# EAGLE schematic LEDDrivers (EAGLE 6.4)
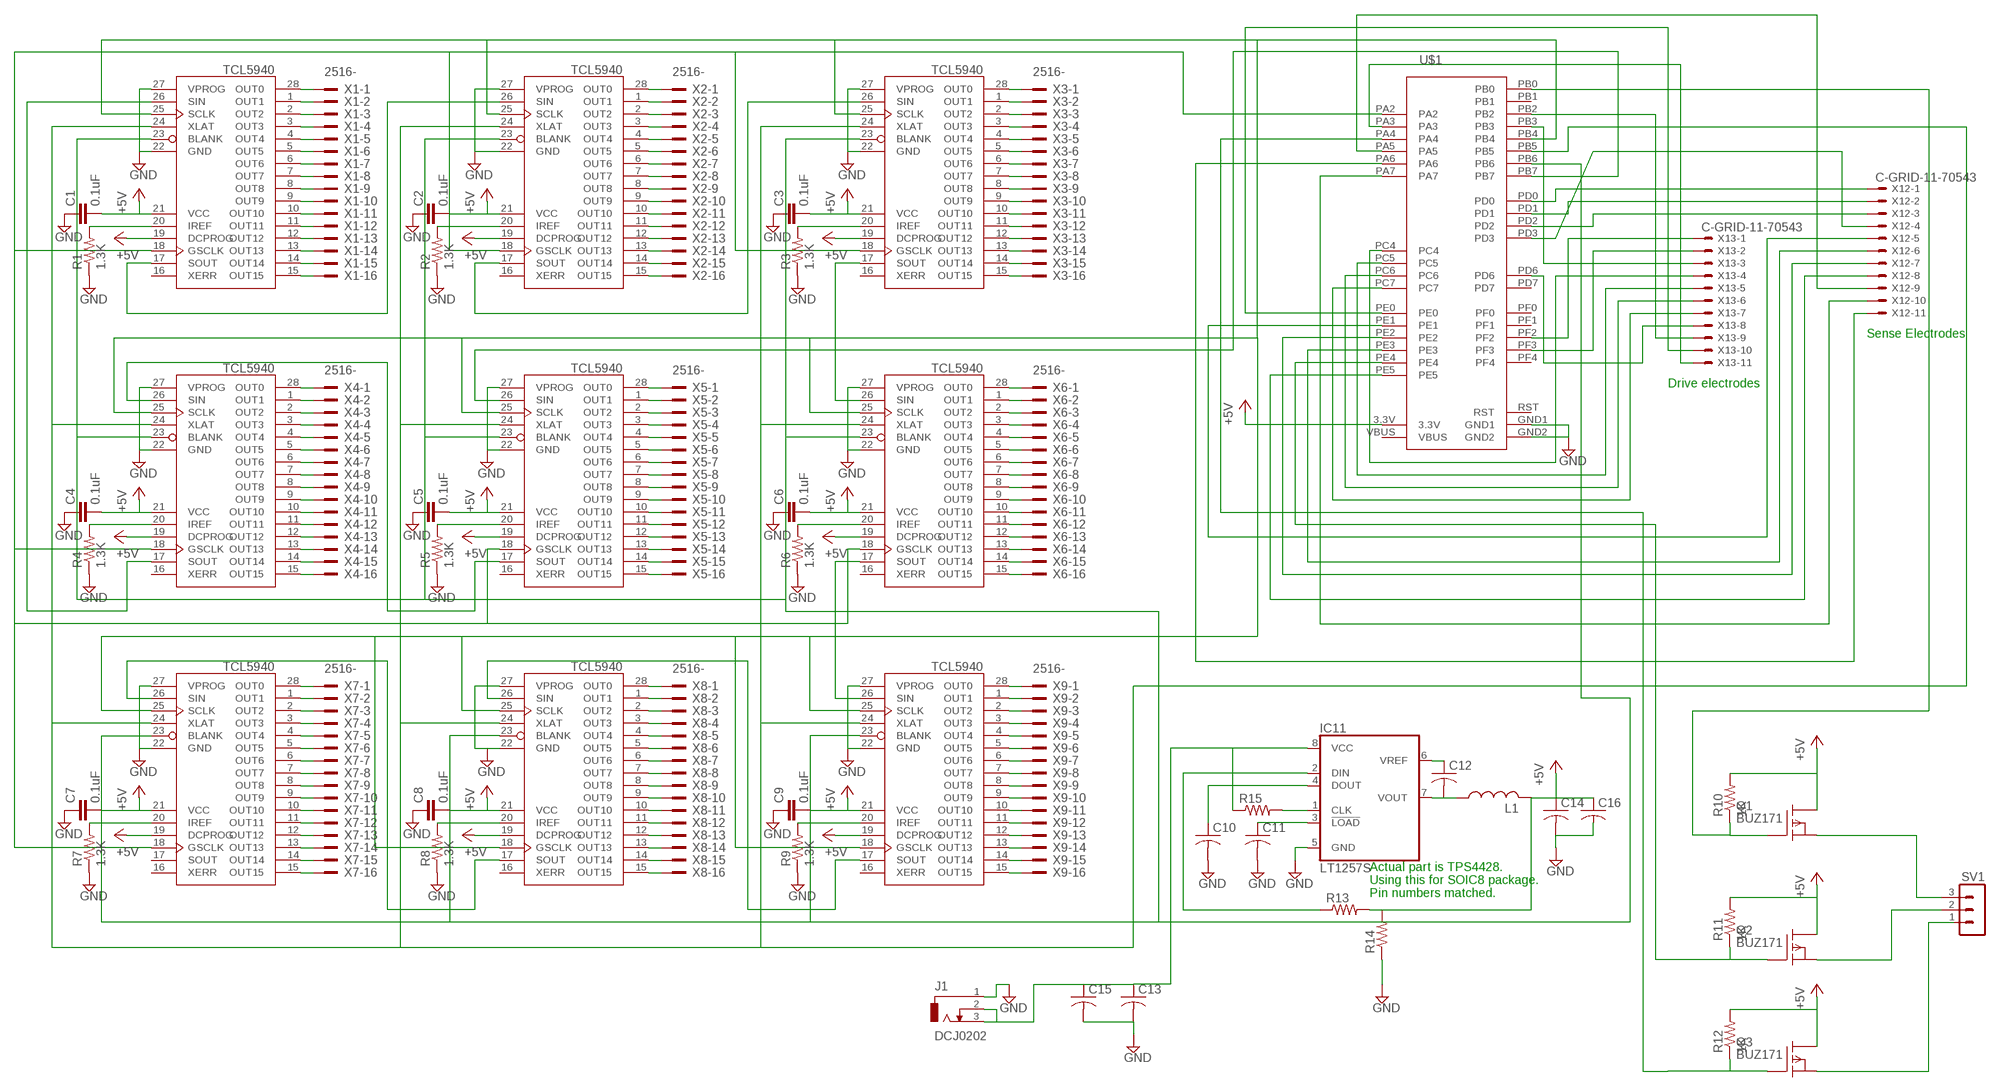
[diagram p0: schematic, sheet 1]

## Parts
C1  0.1uF  C-EU025-024X044  [C025-024X044]
C2  0.1uF  C-EU025-024X044  [C025-024X044]
C3  0.1uF  C-EU025-024X044  [C025-024X044]
C4  0.1uF  C-EU025-024X044  [C025-024X044]
C5  0.1uF  C-EU025-024X044  [C025-024X044]
C6  0.1uF  C-EU025-024X044  [C025-024X044]
C7  0.1uF  C-EU025-024X044  [C025-024X044]
C8  0.1uF  C-EU025-024X044  [C025-024X044]
C9  0.1uF  C-EU025-024X044  [C025-024X044]
C10  C-US025-024X044  [C025-024X044]
C11  C-US025-024X044  [C025-024X044]
C12  C-US025-024X044  [C025-024X044]
C13  C-US025-024X044  [C025-024X044]
C14  C-US025-024X044  [C025-024X044]
C15  C-US025-024X044  [C025-024X044]
C16  C-US025-024X044  [C025-024X044]
IC1  TCL5940  [DIP28]
IC2  TCL5940  [DIP28]
IC3  TCL5940  [DIP28]
IC4  TCL5940  [DIP28]
IC5  TCL5940  [DIP28]
IC6  TCL5940  [DIP28]
IC7  TCL5940  [DIP28]
IC8  TCL5940  [DIP28]
IC9  TCL5940  [DIP28]
IC11  LT1257S  [SOIC8]
J1  DCJ0202  [DCJ0202]
L1  L-US0207/7  [0207/7]
Q1  BUZ171  [TO220]
Q2  BUZ171  [TO220]
Q3  BUZ171  [TO220]
R1  1.3K  R-US_0204/2V  [0204V]
R2  1.3K  R-US_0204/2V  [0204V]
R3  1.3K  R-US_0204/2V  [0204V]
R4  1.3K  R-US_0204/2V  [0204V]
R5  1.3K  R-US_0204/2V  [0204V]
R6  1.3K  R-US_0204/2V  [0204V]
R7  1.3K  R-US_0204/2V  [0204V]
R8  1.3K  R-US_0204/2V  [0204V]
R9  1.3K  R-US_0204/2V  [0204V]
R10  1K  R-US_0204/2V  [0204V]
R11  1K  R-US_0204/2V  [0204V]
R12  1K  R-US_0204/2V  [0204V]
R13  R-US_0204/5  [0204/5]
R14  R-US_0204/5  [0204/5]
R15  R-US_0204/5  [0204/5]
SV1  MA03-1  [MA03-1]
U$1  STELLARIS-LAUNCHPADSTELLARIS-LAUNCHPAD-XL  [LAUNCHPAD-XL]
X1  2516-  [PAK100/2500-16]
X2  2516-  [PAK100/2500-16]
X3  2516-  [PAK100/2500-16]
X4  2516-  [PAK100/2500-16]
X5  2516-  [PAK100/2500-16]
X6  2516-  [PAK100/2500-16]
X7  2516-  [PAK100/2500-16]
X8  2516-  [PAK100/2500-16]
X9  2516-  [PAK100/2500-16]
X12  C-GRID-11-70543  [70543-11]
X13  C-GRID-11-70543  [70543-11]

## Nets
+5V: C1.2 C2.2 C3.2 C4.2 C5.2 C6.2 C7.2 C8.2 C9.2 C14.1 C16.1 IC1.19(DCPROG) IC1.21(VCC) IC2.19(DCPROG) IC2.21(VCC) IC3.19(DCPROG) IC3.21(VCC) IC4.19(DCPROG) IC4.21(VCC) IC5.19(DCPROG) IC5.21(VCC) IC6.19(DCPROG) IC6.21(VCC) IC7.19(DCPROG) IC7.21(VCC) IC8.19(DCPROG) IC8.21(VCC) IC9.19(DCPROG) IC9.21(VCC) L1.2 Q1.2(D) Q2.2(D) Q3.2(D) R10.2 R11.2 R12.2 R13.2 R14.2 U$1.3.3V
GND: C1.1 C2.1 C3.1 C4.1 C5.1 C6.1 C7.1 C8.1 C9.1 C10.2 C11.2 C13.2 C14.2 C15.2 IC1.22(GND) IC1.27(VPROG) IC2.22(GND) IC2.27(VPROG) IC3.22(GND) IC3.27(VPROG) IC4.22(GND) IC4.27(VPROG) IC5.22(GND) IC5.27(VPROG) IC6.22(GND) IC6.27(VPROG) IC7.22(GND) IC7.27(VPROG) IC8.22(GND) IC8.27(VPROG) IC9.22(GND) IC9.27(VPROG) IC11.5(GND) J1.1 R1.1 R2.1 R3.1 R4.1 R5.1 R6.1 R7.1 R8.1 R9.1 R14.1 U$1.GND1 U$1.GND2
N$1: IC1.26(SIN) IC7.17(SOUT)
N$2: IC7.20(IREF) R1.2
N$3: IC1.20(IREF) R2.2
N$4: IC1.28(OUT0) X2.1
N$5: IC1.3(OUT3) X2.4
N$6: IC1.4(OUT4) X2.5
N$7: IC1.5(OUT5) X2.6
N$8: IC1.6(OUT6) X2.7
N$9: IC1.7(OUT7) X2.8
N$10: IC1.8(OUT8) X2.9
N$11: IC1.9(OUT9) X2.10
N$12: IC1.10(OUT10) X2.11
N$13: IC1.11(OUT11) X2.12
N$14: IC1.12(OUT12) X2.13
N$15: IC7.28(OUT0) X1.1
N$16: IC1.13(OUT13) X2.14
N$17: IC1.14(OUT14) X2.15
N$18: IC1.15(OUT15) X2.16
N$19: IC7.1(OUT1) X1.2
N$20: IC7.2(OUT2) X1.3
N$21: IC7.3(OUT3) X1.4
N$22: IC7.4(OUT4) X1.5
N$23: IC7.5(OUT5) X1.6
N$24: IC7.6(OUT6) X1.7
N$25: IC7.7(OUT7) X1.8
N$26: IC7.8(OUT8) X1.9
N$27: IC7.9(OUT9) X1.10
N$28: IC7.10(OUT10) X1.11
N$29: IC7.11(OUT11) X1.12
N$30: IC7.12(OUT12) X1.13
N$31: IC7.13(OUT13) X1.14
N$32: IC7.14(OUT14) X1.15
N$33: IC7.15(OUT15) X1.16
N$34: IC1.1(OUT1) X2.2
N$35: IC1.2(OUT2) X2.3
N$36: IC1.17(SOUT) IC2.26(SIN)
N$37: IC2.20(IREF) R3.2
N$38: IC2.28(OUT0) X3.1
N$39: IC2.3(OUT3) X3.4
N$40: IC2.4(OUT4) X3.5
N$41: IC2.5(OUT5) X3.6
N$42: IC2.6(OUT6) X3.7
N$43: IC2.7(OUT7) X3.8
N$44: IC2.8(OUT8) X3.9
N$45: IC2.9(OUT9) X3.10
N$46: IC2.10(OUT10) X3.11
N$47: IC2.11(OUT11) X3.12
N$48: IC2.12(OUT12) X3.13
N$49: IC2.13(OUT13) X3.14
N$50: IC2.14(OUT14) X3.15
N$51: IC2.15(OUT15) X3.16
N$52: IC2.1(OUT1) X3.2
N$53: IC2.2(OUT2) X3.3
N$54: IC2.17(SOUT) IC5.26(SIN)
N$55: IC3.20(IREF) R4.2
N$56: IC3.28(OUT0) X4.1
N$57: IC3.3(OUT3) X4.4
N$58: IC3.4(OUT4) X4.5
N$59: IC3.5(OUT5) X4.6
N$60: IC3.6(OUT6) X4.7
N$61: IC3.7(OUT7) X4.8
N$62: IC3.8(OUT8) X4.9
N$63: IC3.9(OUT9) X4.10
N$64: IC3.10(OUT10) X4.11
N$65: IC3.11(OUT11) X4.12
N$66: IC3.12(OUT12) X4.13
N$67: IC3.13(OUT13) X4.14
N$68: IC3.14(OUT14) X4.15
N$69: IC3.15(OUT15) X4.16
N$70: IC3.1(OUT1) X4.2
N$71: IC3.2(OUT2) X4.3
N$72: IC3.17(SOUT) IC7.26(SIN)
N$73: IC4.20(IREF) R5.2
N$74: IC4.28(OUT0) X5.1
N$75: IC4.3(OUT3) X5.4
N$76: IC4.4(OUT4) X5.5
N$77: IC4.5(OUT5) X5.6
N$78: IC4.6(OUT6) X5.7
N$79: IC4.7(OUT7) X5.8
N$80: IC4.8(OUT8) X5.9
N$81: IC4.9(OUT9) X5.10
N$82: IC4.10(OUT10) X5.11
N$83: IC4.11(OUT11) X5.12
N$84: IC4.12(OUT12) X5.13
N$85: IC4.13(OUT13) X5.14
N$86: IC4.14(OUT14) X5.15
N$87: IC4.15(OUT15) X5.16
N$88: IC4.1(OUT1) X5.2
N$89: IC4.2(OUT2) X5.3
N$90: IC3.26(SIN) IC4.17(SOUT)
N$91: IC5.20(IREF) R6.2
N$92: IC5.28(OUT0) X6.1
N$93: IC5.3(OUT3) X6.4
N$94: IC5.4(OUT4) X6.5
N$95: IC5.5(OUT5) X6.6
N$96: IC5.6(OUT6) X6.7
N$97: IC5.7(OUT7) X6.8
N$98: IC5.8(OUT8) X6.9
N$99: IC5.9(OUT9) X6.10
N$100: IC5.10(OUT10) X6.11
N$101: IC5.11(OUT11) X6.12
N$102: IC5.12(OUT12) X6.13
N$103: IC5.13(OUT13) X6.14
N$104: IC5.14(OUT14) X6.15
N$105: IC5.15(OUT15) X6.16
N$106: IC5.1(OUT1) X6.2
N$107: IC5.2(OUT2) X6.3
N$108: IC5.17(SOUT) IC9.26(SIN)
N$109: IC6.20(IREF) R7.2
N$110: IC6.28(OUT0) X7.1
N$111: IC6.3(OUT3) X7.4
N$112: IC6.4(OUT4) X7.5
N$113: IC6.5(OUT5) X7.6
N$114: IC6.6(OUT6) X7.7
N$115: IC6.7(OUT7) X7.8
N$116: IC6.8(OUT8) X7.9
N$117: IC6.9(OUT9) X7.10
N$118: IC6.10(OUT10) X7.11
N$119: IC6.11(OUT11) X7.12
N$120: IC6.12(OUT12) X7.13
N$121: IC6.13(OUT13) X7.14
N$122: IC6.14(OUT14) X7.15
N$123: IC6.15(OUT15) X7.16
N$124: IC6.1(OUT1) X7.2
N$125: IC6.2(OUT2) X7.3
N$126: IC1.25(SCLK) IC2.25(SCLK) IC3.25(SCLK) IC4.25(SCLK) IC5.25(SCLK) IC6.25(SCLK) IC7.25(SCLK) IC8.18(GSCLK) IC8.25(SCLK) IC9.18(GSCLK) IC9.25(SCLK) U$1.PB4
N$127: IC8.20(IREF) R8.2
N$128: IC8.28(OUT0) X8.1
N$129: IC8.3(OUT3) X8.4
N$130: IC8.4(OUT4) X8.5
N$131: IC8.5(OUT5) X8.6
N$132: IC8.6(OUT6) X8.7
N$133: IC8.7(OUT7) X8.8
N$134: IC8.8(OUT8) X8.9
N$135: IC8.9(OUT9) X8.10
N$136: IC8.10(OUT10) X8.11
N$137: IC8.11(OUT11) X8.12
N$138: IC8.12(OUT12) X8.13
N$139: IC8.13(OUT13) X8.14
N$140: IC8.14(OUT14) X8.15
N$141: IC8.15(OUT15) X8.16
N$142: IC8.1(OUT1) X8.2
N$143: IC8.2(OUT2) X8.3
N$144: IC6.26(SIN) IC8.17(SOUT)
N$145: IC9.20(IREF) R9.2
N$146: IC9.28(OUT0) X9.1
N$147: IC9.3(OUT3) X9.4
N$148: IC9.4(OUT4) X9.5
N$149: IC9.5(OUT5) X9.6
N$150: IC9.6(OUT6) X9.7
N$151: IC9.7(OUT7) X9.8
N$152: IC9.8(OUT8) X9.9
N$153: IC9.9(OUT9) X9.10
N$154: IC9.10(OUT10) X9.11
N$155: IC9.11(OUT11) X9.12
N$156: IC9.12(OUT12) X9.13
N$157: IC9.13(OUT13) X9.14
N$158: IC9.14(OUT14) X9.15
N$159: IC9.15(OUT15) X9.16
N$160: IC9.1(OUT1) X9.2
N$161: IC9.2(OUT2) X9.3
N$162: IC8.26(SIN) IC9.17(SOUT)
N$163: IC4.26(SIN) U$1.PB7
N$164: U$1.PE1 X12.5
N$165: U$1.PF3 X13.2
N$166: U$1.PF2 X13.1
N$167: U$1.PB3 X13.3
N$168: U$1.PC4 X13.4
N$169: U$1.PC5 X13.5
N$170: U$1.PC6 X13.6
N$171: U$1.PC7 X13.7
N$172: U$1.PD6 X13.8
N$173: U$1.PB2 X13.9
N$174: U$1.PE0 X13.10
N$175: U$1.PA3 X13.11
N$176: Q3.1(G) R12.1 U$1.PA4
N$177: Q2.1(G) R11.1 U$1.PE4
N$178: U$1.PD0 X12.1
N$179: U$1.PD1 X12.2
N$180: U$1.PD2 X12.3
N$181: U$1.PD3 X12.4
N$182: IC1.23(BLANK) IC2.23(BLANK) IC3.23(BLANK) IC4.23(BLANK) IC5.23(BLANK) IC6.23(BLANK) IC7.23(BLANK) IC8.23(BLANK) IC9.23(BLANK) U$1.PB6
N$183: U$1.PE3 X12.6
N$184: U$1.PE2 X12.7
N$185: U$1.PE5 X12.8
N$186: U$1.PA5 X12.9
N$187: U$1.PA7 X12.10
N$188: U$1.PA6 X12.11
N$189: IC1.24(XLAT) IC2.24(XLAT) IC3.24(XLAT) IC4.24(XLAT) IC5.24(XLAT) IC6.24(XLAT) IC7.24(XLAT) IC8.24(XLAT) IC9.24(XLAT) U$1.PB5
N$190: Q1.3(S) SV1.3
N$191: Q2.3(S) SV1.2
N$192: Q3.3(S)
N$193: Q1.1(G) R10.1 U$1.PB0
N$194: C13.1 C15.1 IC11.8(VCC) J1.2 J1.3 R15.1
N$195: C11.1 IC11.3(!LOAD)
N$196: IC1.18(GSCLK) IC2.18(GSCLK) IC3.18(GSCLK) IC4.18(GSCLK) IC5.18(GSCLK) IC6.18(GSCLK) IC7.18(GSCLK) U$1.PA2
N$197: C10.1 IC11.4(DOUT)
N$198: C12.1 IC11.6(VREF)
N$199: C12.2 IC11.7(VOUT) L1.1
N$200: IC11.2(DIN) R13.1
N$201: IC11.1(CLK) R15.2
Unconnected: C16.2 IC1.16(XERR) IC2.16(XERR) IC3.16(XERR) IC4.16(XERR) IC5.16(XERR) IC6.16(XERR) IC6.17(SOUT) IC7.16(XERR) IC8.16(XERR) IC9.16(XERR) SV1.1 U$1.PB1 U$1.PD7 U$1.PF0 U$1.PF1 U$1.PF4

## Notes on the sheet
- Sense Electrodes
- Drive electrodes
- Actual part is TPS4428. 
  Using this for SOIC8 package. 
  Pin numbers matched.

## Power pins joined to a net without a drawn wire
RST: U$1.RST
VBUS: U$1.VBUS

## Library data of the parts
C1-C9 = rcl:C-EU: CAPACITOR, European symbol
C10-C16 = resistor:C-US: CAPACITOR, American symbol
IC1-IC9 = tcl5940(1):TCL5940: 16-Channel 12-Bit LED Driver
IC11 = linear-technology:LT1257: Complete Single Supply 12-Bit Voltage Output DAC Source: http://www.linear.com/pc/downloadDocument.do?navId=H0,C1,C1155,C1005,C1156,P1425,D3414; OC_FARNELL: unknown; OC_NEWARK: unknown
J1 = con-jack:DCJ0202: DC POWER JACK Source: DCJ0202.pdf; OC_FARNELL: unknown; OC_NEWARK: unknown
L1 = rcl:L-US: INDUCTOR, American symbol
Q1-Q3 = transistor-fet:BUZ171: P-Channel Enhancement MOSFET -50V; 7A; 0,4Ohm
R1-R15 = resistor:R-US_: RESISTOR, American symbol
SV1 = con-lstb:MA03-1: PIN HEADER; OC_FARNELL: unknown; OC_NEWARK: unknown
U$1 = StellarisLaunchPad_Fred:STELLARIS-LAUNCHPAD
X1-X9 = con-3m:2516-: 3M (TM) Pak 100 4-Wall Header Source: 3M; OC_FARNELL: unknown; OC_NEWARK: unknown
X12 X13 = con-molex:C-GRID-11: CONNECTOR wire to board 2.54 mm (0.100") pitch header; OC_FARNELL: unknown; OC_NEWARK: unknown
